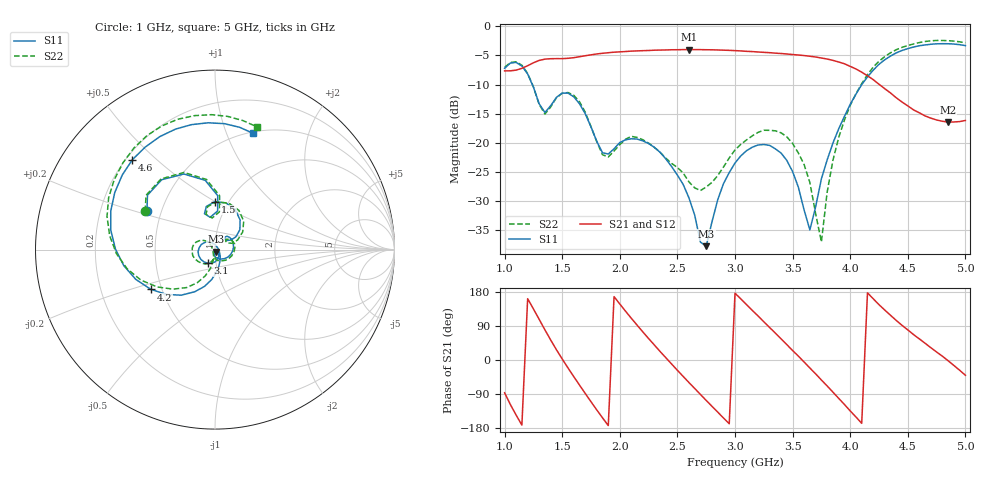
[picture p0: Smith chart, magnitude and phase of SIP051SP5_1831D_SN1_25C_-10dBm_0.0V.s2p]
# GHz  S  dB  R  50
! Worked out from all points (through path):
!   81 points, 1 GHz to 5 GHz, reference 50 ohm
!   highest |S21| = -4.00 dB at 2.6 GHz (marker M1); lowest = -16.4 dB at 4.85 GHz (marker M2)
!   lowest |S11| = -37.7 dB at 2.75 GHz (marker M3), VSWR 1.03, Z = 50.5 - j1.22 ohm
!   |S11| at or under -10 dB: 1.241 GHz to 4.1 GHz (2.86 GHz wide, 107 % of centre)
!   |S22| runs from -37.0 to -2.4 dB; largest |S21 - S12| = 0.004
!   S11 on the Smith chart (normalised r, x): 1 GHz: 0.42, +0.22; 1.5 GHz: 0.87, +0.50; 3.1 GHz: 0.91, -0.14; 4.2 GHz: 0.44, -0.23; 4.6 GHz: 0.23, +0.42; 5 GHz: 0.51, +1.25
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1  -7.20 150.3  -7.65 -86.5  -7.64 -86.7  -7.04 151.2
1.2  -8.18 98.1  -6.77 161.8  -6.77 162.2  -8.09 97.0
1.35  -14.79 98.5  -5.64 79.6  -5.63 79.5  -15.06 95.2
1.5  -11.46 90.0  -5.56 2.6  -5.55 2.9  -11.50 88.1
1.7  -15.00 38.8  -5.06 -88.3  -5.06 -88.3  -14.75 32.5
1.95  -21.01 51.7  -4.45 167.2  -4.46 167.1  -21.39 42.7
2.15  -19.35 19.4  -4.23 92.1  -4.22 92.2  -19.07 5.2
2.35  -21.62 -30.7  -4.09 22.4  -4.09 22.6  -21.61 -45.7
2.6  -29.43 -95.1  -4.00 -59.4  -4.01 -59.4  -26.69 -87.4
2.75  -37.72 -68.8  -4.03 -106.6  -4.03 -106.5  -27.57 -94.0
3  -23.46 -88.4  -4.18 176.3  -4.18 176.3  -21.21 -115.9
3.1  -21.35 -117.7  -4.30 146.0  -4.29 146.2  -19.50 -134.2
3.35  -21.02 173.5  -4.61 70.9  -4.61 70.8  -17.93 175.3
3.65  -34.93 25.7  -5.14 -21.2  -5.15 -21.0  -26.82 131.1
3.7  -30.98 -27.8  -5.28 -36.5  -5.28 -36.5  -32.15 139.5
3.75  -26.16 -53.4  -5.45 -52.8  -5.44 -52.7  -36.99 -142.6
3.9  -17.60 -87.7  -6.13 -101.2  -6.13 -101.2  -19.09 -104.0
4.2  -7.53 -148.2  -9.16 161.6  -9.22 161.1  -7.00 -157.7
4.35  -5.12 179.7  -11.45 118.0  -11.48 117.8  -4.56 172.6
4.6  -3.35 132.6  -14.85 55.7  -14.90 55.5  -2.80 128.4
4.85  -3.00 93.1  -16.43 -2.0  -16.41 -2.0  -2.48 91.5
5  -3.33 71.8  -16.16 -40.2  -16.17 -40.7  -2.83 70.9
